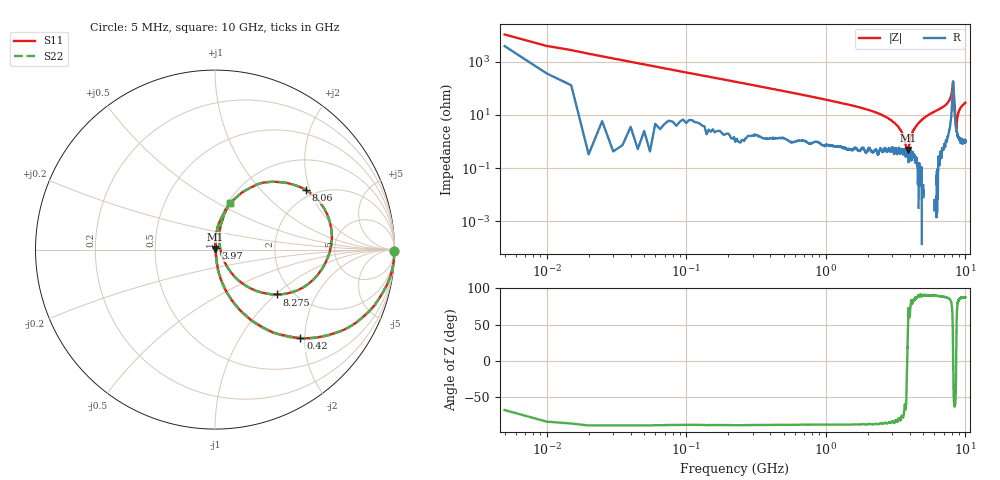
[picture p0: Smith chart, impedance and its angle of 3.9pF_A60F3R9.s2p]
! Amotech Co.,Ltd.
! http://www.amotech.co.kr/
! Part Number: A60F3R9
! These Parameters are Measured in Series Mode Connection
! Operation Temp=25[degC], DC Bias Voltage=0[V]
! Freq. Start=5[MHz] Stop=10[GHz], 2000[Steps]
! Date: Monday, July 20, 2020, 03:25:01
# GHZ S RI R 50.000000
!Freq.(Hz) S11(Real) S11(Imag) S21(Real) S21(Imag) S12(Real) S12(Imag) S22(Real) S22(Imag)
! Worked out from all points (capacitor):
!   2000 points, 5 MHz to 10 GHz, reference 50 ohm
!   read as one part in series: C = 3.98 pF near 55 MHz
!   lowest |Z| = 481 mohm at 3.895 GHz (marker M1)
!   series resonance near 3.831 GHz, so ESL is about 430 pH
!   S11 on the Smith chart (normalised r, x): 5 MHz: open; 420 MHz: 1.03, -1.90; 3.97 GHz: 1.01, +0.02; 8.06 GHz: 1.79, +1.87; 8.275 GHz: 1.67, -1.02; 10 GHz: 1.02, +0.58
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0.005  0.9966 -0.00856  0.00344 0.00856  0.00344 0.00856  0.9966 -0.00856
0.065  0.9734 -0.1584  0.0266 0.1584  0.0266 0.1584  0.9734 -0.1584
0.12  0.9148 -0.2715  0.0852 0.2715  0.0852 0.2715  0.9148 -0.2715
0.42  0.4754 -0.492  0.5246 0.492  0.5246 0.492  0.4754 -0.492
0.87  0.1683 -0.3634  0.8317 0.3634  0.8317 0.3634  0.1683 -0.3634
1.675  0.0446 -0.1941  0.9554 0.1941  0.9554 0.1941  0.0446 -0.1941
3.34  0.00692 -0.0323  0.9931 0.0323  0.9931 0.0323  0.00692 -0.0323
3.6  0.00371 -0.0159  0.9963 0.0159  0.9963 0.0159  0.00371 -0.0159
3.77  0.00325 -0.00511  0.9967 0.00511  0.9967 0.00511  0.00325 -0.00511
3.895  0.00258 0.00405  0.9974 -0.00405  0.9974 -0.00405  0.00258 0.00405
3.97  0.0038 0.0077  0.9962 -0.0077  0.9962 -0.0077  0.0038 0.0077
4.235  0.00348 0.0267  0.9965 -0.0267  0.9965 -0.0267  0.00348 0.0267
5.005  0.00567 0.0736  0.9943 -0.0736  0.9943 -0.0736  0.00567 0.0736
6.67  0.0351 0.1736  0.9649 -0.1736  0.9649 -0.1736  0.0351 0.1736
7.71  0.1414 0.3109  0.8586 -0.3109  0.8586 -0.3109  0.1414 0.3109
8.06  0.5058 0.3321  0.4942 -0.3321  0.4942 -0.3321  0.5058 0.3321
8.16  0.6483 0.0336  0.3517 -0.0336  0.3517 -0.0336  0.6483 0.0336
8.275  0.3447 -0.2497  0.6553 0.2497  0.6553 0.2497  0.3447 -0.2497
8.335  0.1946 -0.2142  0.8054 0.2142  0.8054 0.2142  0.1946 -0.2142
8.6  0.0291 0.00558  0.9709 -0.00558  0.9709 -0.00558  0.0291 0.00558
8.995  0.0313 0.1349  0.9687 -0.1349  0.9687 -0.1349  0.0313 0.1349
10  0.086 0.2623  0.914 -0.2623  0.914 -0.2623  0.086 0.2623
